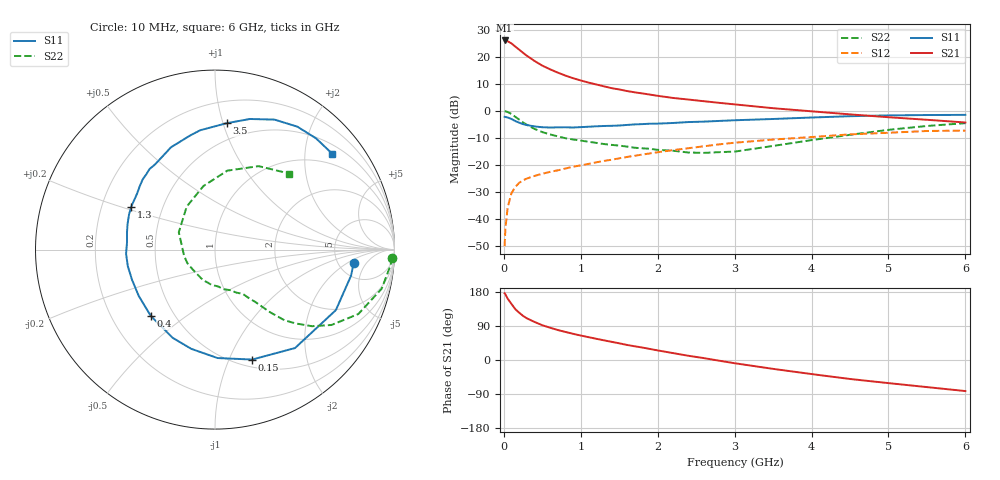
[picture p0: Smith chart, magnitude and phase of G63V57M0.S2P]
! SIEMENS Small Signal Semiconductors
! BFG193
! Si NPN RF Bipolar Junction Transistor in SOT223
! VCE = 3.5 V  IC = 7 mA
! Common Emitter S-Parameters:  August  1996
# GHz  S  MA  R  50
!  f  S11  S21  S12  S22
! GHz  MAG  ANG  MAG  ANG  MAG  ANG  MAG  ANG
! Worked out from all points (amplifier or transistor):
!   36 points, 10 MHz to 6 GHz, reference 50 ohm
!   highest |S21| = 26.1 dB at 10 MHz (marker M1)
!   |S21| within 3 dB of that: start of sweep to 181.1 MHz
!   unconditionally stable (mu >= 1): 986.7 MHz to 2.533 GHz
!   at 250 MHz: K = 0.42, MSG = 23.6 dB, |S12| = -25.7 dB
!   at 1.4 GHz: K = 1.08, MAG = 11.5 dB, |S12| = -18.1 dB
!   at 6 GHz: K = 0.88, MSG = 1.5 dB, |S12| = -7.3 dB
!   S11 on the Smith chart (normalised r, x): 10 MHz: 6.95, -2.60; 150 MHz: 0.58, -1.22; 400 MHz: 0.37, -0.37; 1.3 GHz: 0.33, +0.22; 3.5 GHz: 0.36, +1.03; 6 GHz: 0.71, +2.62
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0.01  0.7763 -5.5  20.22 176.0  0.0031 92.0  0.9889 -2.6
0.02  0.7718 -10.9  20.21 173.4  0.0065 87.7  0.9805 -5.4
0.05  0.7531 -26.6  19.55 161.7  0.0163 75.7  0.9539 -13.2
0.1  0.7068 -50.9  17.79 147.7  0.0299 66.8  0.8757 -24.2
0.15  0.6467 -71.3  15.5 133.9  0.039 58.1  0.7731 -32.9
0.2  0.6043 -88.7  13.64 124.7  0.0464 53.1  0.6887 -38.3
0.25  0.5684 -103.5  11.91 116.4  0.0517 49.1  0.6089 -42.5
0.3  0.5452 -115.6  10.52 109.9  0.0557 47.2  0.5518 -45.5
0.4  0.5143 -134.0  8.404 100.3  0.0623 44.7  0.462 -48.8
0.5  0.4974 -148.6  6.905 91.8  0.0682 43.7  0.404 -50.8
0.6  0.492 -160.1  5.906 85.3  0.074 43.9  0.3661 -52.5
0.7  0.4945 -169.3  5.132 79.2  0.0789 44.3  0.3368 -54.6
0.9  0.4918 175.4  4.035 69.1  0.0921 44.3  0.2948 -57.6
1.1  0.508 163.5  3.349 60.3  0.1041 44.2  0.268 -63.5
1.3  0.5244 152.9  2.855 52.0  0.118 43.5  0.2427 -68.9
1.6  0.5482 139.9  2.334 39.8  0.1398 41.0  0.218 -80.7
2.2  0.5968 119.1  1.737 18.2  0.1872 33.3  0.1825 -111.7
2.8  0.651 102.2  1.409 -1.9  0.2395 22.8  0.1716 -154.3
3.5  0.7074 84.7  1.121 -23.4  0.2939 7.4  0.2238 154.3
4.5  0.7965 65.4  0.861 -50.1  0.3667 -12.7  0.36 100.3
5.5  0.8374 47.7  0.684 -71.5  0.4238 -37.7  0.5247 62.4
6  0.8434 39.4  0.609 -82.0  0.431 -52.0  0.5921 45.7
